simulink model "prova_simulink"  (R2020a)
settings: Solver=VariableStepAuto  StartTime=0.0  StopTime=10.0  RelTol=1e-3
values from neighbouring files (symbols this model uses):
  a = 3    [prova_script.m]
libraries: simulink x1

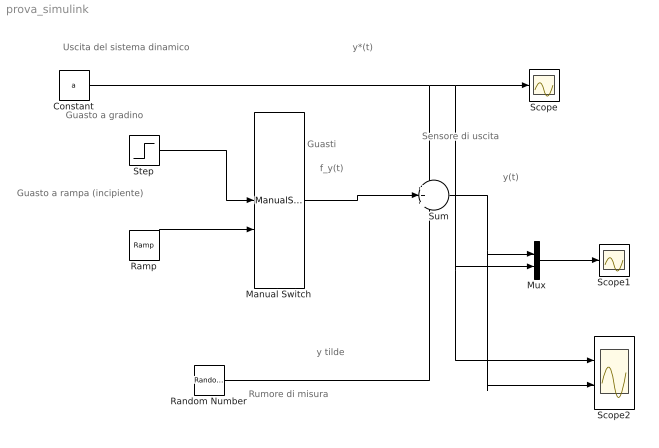
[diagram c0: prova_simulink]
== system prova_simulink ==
  note: Rumore di misura
  note: y tilde
  note: f_y(t)
  note: y(t)
  note: Guasto a rampa (incipiente)
  note: Guasto a gradino
  note: Guasti
  note: Sensore di uscita
  note: y*(t)
  note: Uscita del sistema dinamico
  Constant : Constant  Value=a  SampleTime=0
  Manual Switch : ManualSwitch
  Mux : Mux  Inputs=2
  Ramp : simulink/Sources/Ramp  slope=1  start=5  InitialOutput=0
  Random Number : RandomNumber  Variance=(3)^2  SampleTime=0.1
  Scope : Scope
  Scope1 : Scope
  Scope2 : Scope  NumInputPorts=2
  Step : Step  Time=5  SampleTime=0
  Sum : Sum  Inputs=+++
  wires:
  Constant/1 -> Scope2/1, Mux/2, Scope/1, Sum/1
  Manual Switch/1 -> Sum/2
  Step/1 -> Manual Switch/1
  Ramp/1 -> Manual Switch/2
  Sum/1 -> Scope2/2, Mux/1
  Mux/1 -> Scope1/1
  Random Number/1 -> Sum/3
